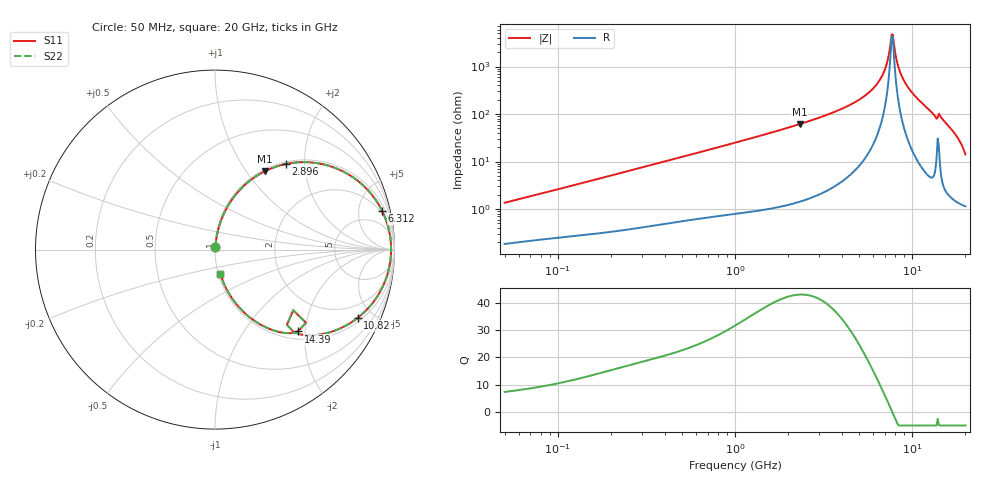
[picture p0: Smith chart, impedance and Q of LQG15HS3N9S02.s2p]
!Murata Part Number: LQG15HS3N9S02
!These Parameters are Measured in Series Mode Connection
!  o--[Z]--o
!Port1  Port2
!  o-------o
!Freq. Start=50[MHz] Stop=20[GHz], 401[Steps]
# Hz S RI R 50
!Freq.(Hz) S11(Real) S11(Imag) S21(Real) S21(Imag) S12(Real) S12(Imag) S22(Real) S22(Imag)
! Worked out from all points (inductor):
!   401 points, 50 MHz to 20 GHz, reference 50 ohm
!   read as one part in series: L = 4.23 nH near 51.52 MHz
!   highest Q = 43 at 2.314 GHz (marker M1), where L = 4.21 nH
!   self-resonance near 7.668 GHz
!   S11 on the Smith chart (normalised r, x): 50 MHz: 1.00, +0.03; 2.896 GHz: 1.04, +1.61; 6.312 GHz: 1.68, +8.40; 10.82 GHz: 1.20, -4.07; 14.39 GHz: 1.16, -1.84; 20 GHz: 1.02, -0.28
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5e7  0.00203 0.0134  0.998 -0.0134  0.998 -0.0134  0.00203 0.0134
1.364002e8  0.00403 0.0348  0.996 -0.0348  0.996 -0.0348  0.00403 0.0348
3.721004e8  0.0132 0.0917  0.9868 -0.0917  0.9868 -0.0917  0.0132 0.0917
1e9  0.0649 0.231  0.9351 -0.231  0.9351 -0.231  0.0649 0.231
2.313601e9  0.2773 0.4362  0.7227 -0.4362  0.7227 -0.4362  0.2773 0.4362
2.728004e9  0.3613 0.4687  0.6387 -0.4687  0.6387 -0.4687  0.3613 0.4687
2.896447e9  0.3963 0.4773  0.6037 -0.4773  0.6037 -0.4773  0.3963 0.4773
4.677679e9  0.7383 0.422  0.2617 -0.422  0.2617 -0.422  0.7383 0.422
6.311513e9  0.9311 0.2162  0.0689 -0.2162  0.0689 -0.2162  0.9311 0.2162
7.009217e9  0.9688 0.1101  0.0312 -0.1101  0.0312 -0.1101  0.9688 0.1101
7.442007e9  0.9793 0.0433  0.0207 -0.0433  0.0207 -0.0433  0.9793 0.0433
7.668323e9  0.9811 0.00864  0.0189 -0.00864  0.0189 -0.00864  0.9811 0.00864
7.784049e9  0.981 -0.00895  0.019 0.00895  0.019 0.00895  0.981 -0.00895
8.389408e9  0.9707 -0.0986  0.0293 0.0986  0.0293 0.0986  0.9707 -0.0986
8.774992e9  0.956 -0.1527  0.044 0.1527  0.044 0.1527  0.956 -0.1527
9.600142e9  0.9059 -0.258  0.0941 0.258  0.0941 0.258  0.9059 -0.258
1.082228e10  0.7947 -0.3806  0.2053 0.3806  0.2053 0.3806  0.7947 -0.3806
1.276073e10  0.5607 -0.4763  0.4393 0.4763  0.4393 0.4763  0.5607 -0.4763
1.438523e10  0.4635 -0.4559  0.5365 0.4559  0.5365 0.4559  0.4635 -0.4559
1.527346e10  0.3289 -0.4513  0.6711 0.4513  0.6711 0.4513  0.3289 -0.4513
1.721783e10  0.1542 -0.3428  0.8458 0.3428  0.8458 0.3428  0.1542 -0.3428
2e10  0.0303 -0.1355  0.9697 0.1355  0.9697 0.1355  0.0303 -0.1355
